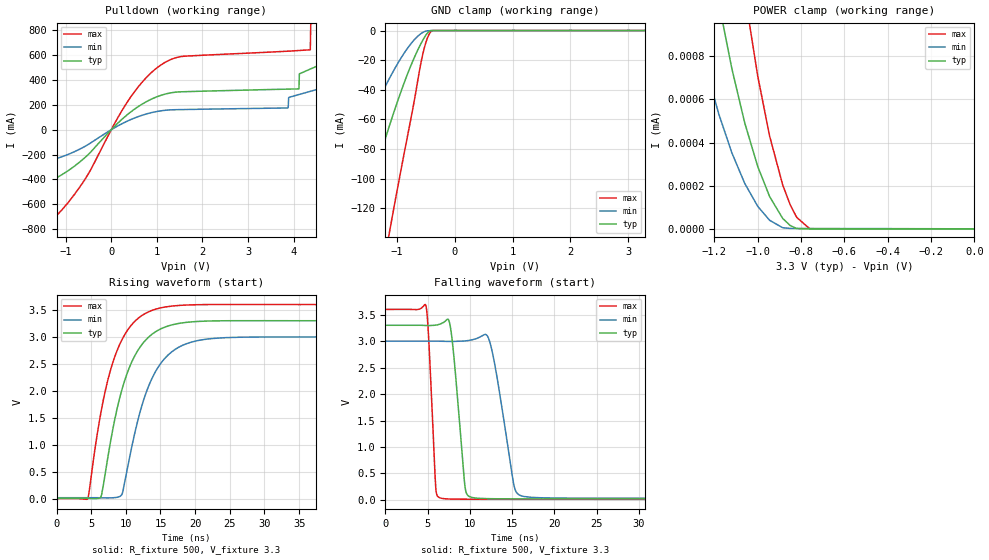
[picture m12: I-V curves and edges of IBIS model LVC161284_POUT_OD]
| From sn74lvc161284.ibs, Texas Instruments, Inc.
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[Model]   LVC161284_POUT_OD
Model_type  Open_drain
Enable   Active-Low
Vref =   3.3
Rref =   500
Cref =   50p
Vmeas =   1.5
| variable   typ   min   max
C_comp   5.54pF   4.51pF   6.31pF
| C_pulldown   9.06pF   6.12pF   13.46pF
| C_tri-state   5.54pF   4.51pF   6.31pF
[Temperature Range]   40   100   -40
| Ambient temperature   25   85   -40
[Voltage range]   3.3   3   3.6
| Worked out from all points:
|   slope of the pulldown table from 0 to 0.495 V, typ, clamps not added: 3.07 ohm
|   GND clamp passes 1 mA (typ) near -0.46 V on its own axis
|   rising waveform, R_fixture 500, V_fixture 3.3: 20-80 % time 3.98ns typ, 4.18ns min, 3.85ns max; typ from 0.017 V to 3.3 V
|   falling waveform, R_fixture 500, V_fixture 3.3: 20-80 % time 1.04ns typ, 1.74ns min, 624ps max; typ from 3.3 V to 0.019 V
[GND Clamp]
| LVC161284_POUT_OD
|   Voltage   I(typ)   I(min)   I(max)
-5.5V     -749.3mA   -479.4mA   -1.295A
-2.285V   -225.9mA   -135.4mA   -414.8mA
-1.71V    -141.1mA   -80.56mA   -270.3mA
-1.645V   -131.9mA   -74.7mA    -254.5mA
-1.395V   -97.8mA    -53.05mA   -195.4mA
-1.125V   -63.49mA   -31.82mA   -134.9mA
-840mV    -31.55mA   -13.16mA   -75.59mA
-710mV    -19.07mA   -6.611mA   -49.21mA
-575mV    -8.028mA   -1.804mA   -19.73mA
-485mV    -2.272mA   -257.2uA   -6.247mA
-405mV    -3.226uA   -76.63uA   -485.3uA
3.3V      9.008pA    1.839nA    5.521pA
[POWER Clamp]
| LVC161284_POUT_OD
|   Voltage   I(typ)   I(min)   I(max)
-5.5V     123.6uA    84.5uA     191uA
-1.3V     1.809uA    996.7nA    3.367uA
-1.24V    1.403uA    747nA      2.685uA
-1.18V    1.048uA    532.4nA    2.077uA
-1.12V    743.9nA    353.5nA    1.545uA
-1.06V    490.5nA    210.7nA    1.087uA
-1V       288.8nA    104.5nA    706.8nA
-945mV    149.4nA    39.89nA    429.1nA
-885mV    48.88nA    5.745nA    204.4nA
-820mV    1.866nA    2.294nA    53.4nA
-760mV    143.3pA    2.238nA    816.5pA
-95.1fV   9.008pA    644.5pA    9.42pA
[Pulldown]
| LVC161284_POUT_OD
|   Voltage   I(typ)   I(min)   I(max)
-5.5V     -519.7mA   -307.6mA   -940.8mA
-1.625V   -455mA     -270.1mA   -819.6mA
-705mV    -263.7mA   -158.6mA   -468.6mA
610mV     190.5mA    108mA      353mA
1.425V    302.7mA    161.3mA    580mA
3.87V     326.6mA    175.1mA    631.7mA
4.115V    328.5mA    283mA      637.2mA
4.125V    449.6mA    284mA      637.4mA
4.365V    488mA      308.8mA    643mA
4.375V    489.6mA    309.9mA    848.3mA
6.51V     834.7mA    534.6mA    1.434A
11V       1.573A     1.016A     2.641A
[Ramp]
| LVC161284_POUT_OD
| variable   typ   min   max
dV/dt_r   1.97/3.98E-09   1.79/4.18E-09   2.16/3.86E-09
dV/dt_f   2.04/1.08E-09   1.86/1.83E-09   2.21/6.44E-10
R_load = 500
[Rising Waveform]
| LVC161284_POUT_OD
R_fixture =   500
C_fixture =   0
L_fixture =   0
V_fixture =   3.3
V_fixture_min = 3
V_fixture_max = 3.6
|   Time   V(typ)   V(min)   V(max)
0s        17.15mV    26.87mV    10.24mV
4.48ns    15.91mV    26.86mV    8.418mV
6.39ns    41.52mV    25.84mV    1.593V
7.81ns    1.077V     24.56mV    2.398V
9.455ns   2.035V     95.42mV    2.955V
10.96ns   2.57V      1.034V     3.246V
12.76ns   2.93V      1.911V     3.433V
15.71ns   3.188V     2.617V     3.557V
20.05ns   3.286V     2.926V     3.598V
50ns      3.301V     3.001V     3.6V
[Falling Waveform]
| LVC161284_POUT_OD
R_fixture =   500
C_fixture =   0
L_fixture =   0
V_fixture =   3.3
V_fixture_min = 3
V_fixture_max = 3.6
|   Time   V(typ)   V(min)   V(max)
0s        3.3V       3V         3.6V
4.775ns   3.296V     3V         3.676V
5.95ns    3.302V     3V         239mV
6.405ns   3.32V      2.999V     42.1mV
7.675ns   3.278V     2.996V     16.78mV
9.38ns    299.8mV    3.003V     13.39mV
9.975ns   60.88mV    3.016V     13.07mV
12.31ns   23.71mV    3.009V     12.4mV
15.91ns   20.25mV    88.37mV    11.95mV
50ns      19.06mV    30.02mV    11.34mV
